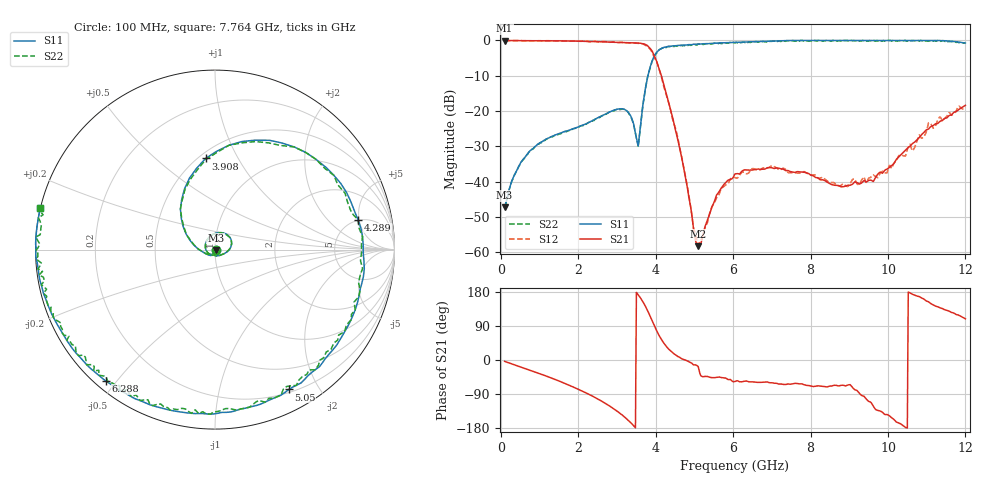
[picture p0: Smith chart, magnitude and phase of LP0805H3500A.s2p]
!	AVX	THIN	FILM	OPERATION
!	LP0805	High	Performance	Low	Pass	Filter	P/N	LP0805H3500ASTR
!	28	June	2017
#	MHz	S	dB	R	50
!	Frq	S11(dB)	S11(deg)	S21(dB)	S21(deg)	S12(dB)	S12(deg)	S22(dB)	S22(deg)
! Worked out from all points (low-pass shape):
!   501 points, 100 MHz to 12 GHz, reference 50 ohm
!   highest |S21| = -0.02 dB at 100 MHz (marker M1); lowest = -58.3 dB at 5.098 GHz (marker M2)
!   |S21| within 3 dB of the highest: start of sweep to 3.91 GHz
!   lowest |S11| = -47.3 dB at 100 MHz (marker M3), VSWR 1.01, Z = 50.4 - j0.217 ohm
!   |S11| at or under -10 dB: start of sweep to 3.802 GHz
!   |S22| runs from -47.3 to 0.0 dB; largest |S21 - S12| = 0.042
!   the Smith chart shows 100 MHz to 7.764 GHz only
!   S11 on the Smith chart (normalised r, x): 100 MHz: 1.01, -0.00; 3.908 GHz: 0.54, +0.74; 4.289 GHz: 4.86, +4.82; 5.05 GHz: 0.23, -1.63; 6.288 GHz: 0.03, -0.47; 7.764 GHz: -0.00, +0.12
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100  -47.33 -30.1  -0.02 -3.6  -0.01 -3.7  -47.33 -30.2
766.4  -31.19 -114.5  -0.08 -27.4  -0.08 -27.3  -31.19 -114.6
2099.2  -24.05 145.3  -0.22 -81.8  -0.20 -81.6  -24.15 145.3
2884.6  -19.93 69.9  -0.50 -126.3  -0.39 -126.4  -19.93 69.9
3265.4  -20.06 20.9  -0.63 -156.6  -0.67 -157.2  -20.06 20.7
3551  -29.91 -103.2  -0.72 172.0  -0.79 171.1  -30.11 -103.3
3908  -5.84 95.9  -2.97 104.3  -3.27 102.0  -5.94 95.9
4074.6  -2.82 52.2  -7.52 67.5  -7.59 66.6  -2.82 52.2
4288.8  -1.79 11.9  -15.57 34.4  -15.93 38.0  -1.79 11.7
4669.6  -1.36 -32.3  -33.01 3.5  -32.83 6.3  -1.36 -32.3
5050.4  -1.10 -62.2  -57.47 -13.6  -55.67 -16.5  -1.30 -62.3
5098  -1.01 -65.6  -58.32 -16.9  -57.98 -28.1  -1.01 -65.6
5597.8  -0.74 -95.6  -43.48 -45.3  -44.31 -49.8  -0.74 -95.6
6050  -0.51 -118.3  -37.82 -56.8  -38.87 -57.1  -0.71 -118.5
6288  -0.43 -129.7  -36.69 -56.0  -37.33 -59.8  -0.53 -129.8
7763.6  0.00 166.7  -37.29 -62.9  -37.50 -65.5  0.00 166.7
8049.2  0.00 153.7  -38.31 -69.5  -38.11 -69.8  -0.20 153.7
9144  0.00 95.8  -40.06 -78.5  -39.27 -82.8  -0.10 95.8
10024.6  0.00 40.4  -36.11 -146.3  -35.68 -153.8  0.00 40.3
10952.8  0.00 -21.0  -25.77 158.8  -26.80 169.0  0.00 -21.1
11500.2  -0.12 -58.8  -21.99 131.6  -21.73 135.6  -0.32 -58.8
12000  -0.72 -93.2  -18.39 108.6  -18.87 110.8  -0.82 -93.4
